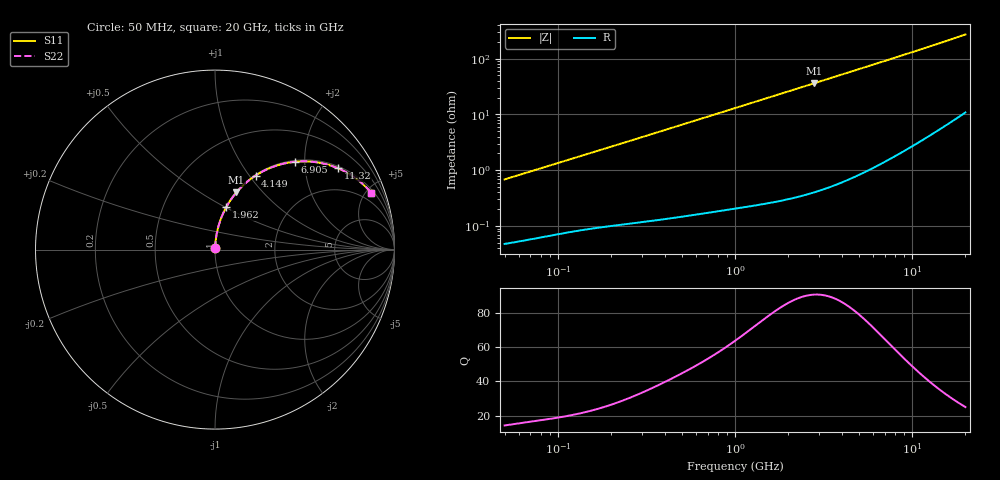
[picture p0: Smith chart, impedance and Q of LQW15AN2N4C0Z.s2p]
!Murata Part Number: LQW15AN2N4C0Z
!These Parameters are Measured in Series Mode Connection
!  o--[Z]--o
!Port1  Port2
!  o-------o
!Freq. Start=50[MHz] Stop=20[GHz], 401[Steps]
# Hz S RI R 50
!Freq.(Hz) S11(Real) S11(Imag) S21(Real) S21(Imag) S12(Real) S12(Imag) S22(Real) S22(Imag)
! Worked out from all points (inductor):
!   401 points, 50 MHz to 20 GHz, reference 50 ohm
!   read as one part in series: L = 2.16 nH near 51.52 MHz
!   highest Q = 90.4 at 2.811 GHz (marker M1), where L = 2.06 nH
!   S11 on the Smith chart (normalised r, x): 50 MHz: 1.00, +0.01; 1.962 GHz: 1.01, +0.51; 4.149 GHz: 1.01, +1.07; 6.905 GHz: 1.03, +1.79; 11.32 GHz: 1.07, +2.97; 20 GHz: 1.22, +5.43
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5e7  0.000523 0.00682  0.9995 -0.00682  0.9995 -0.00682  0.000523 0.00682
5.152053e7  0.000533 0.00703  0.9995 -0.00703  0.9995 -0.00703  0.000533 0.00703
1.364002e8  0.00117 0.0181  0.9988 -0.0181  0.9988 -0.0181  0.00117 0.0181
2.33884e8  0.00201 0.0307  0.998 -0.0307  0.998 -0.0307  0.00201 0.0307
3.721004e8  0.00364 0.0485  0.9964 -0.0485  0.9964 -0.0485  0.00364 0.0485
6.285508e8  0.00825 0.081  0.9918 -0.081  0.9918 -0.081  0.00825 0.081
1e9  0.0185 0.1271  0.9815 -0.1271  0.9815 -0.1271  0.0185 0.1271
1.411297e9  0.0345 0.1761  0.9655 -0.1761  0.9655 -0.1761  0.0345 0.1761
1.962148e9  0.063 0.2372  0.937 -0.2372  0.937 -0.2372  0.063 0.2372
2.728004e9  0.1134 0.3116  0.8866 -0.3116  0.8866 -0.3116  0.1134 0.3116
2.810964e9  0.1195 0.3189  0.8805 -0.3189  0.8805 -0.3189  0.1195 0.3189
3.415248e9  0.1661 0.3667  0.8339 -0.3667  0.8339 -0.3667  0.1661 0.3667
4.149438e9  0.2266 0.4128  0.7734 -0.4128  0.7734 -0.4128  0.2266 0.4128
5.433528e9  0.3337 0.465  0.6663 -0.465  0.6663 -0.465  0.3337 0.465
6.905011e9  0.4467 0.4896  0.5533 -0.4896  0.5533 -0.4896  0.4467 0.4896
7.442007e9  0.4839 0.4917  0.5161 -0.4917  0.5161 -0.4917  0.4839 0.4917
9.178299e9  0.5877 0.4828  0.4123 -0.4828  0.4123 -0.4828  0.5877 0.4828
1.131968e10  0.6843 0.4535  0.3157 -0.4535  0.3157 -0.4535  0.6843 0.4535
1.314879e10  0.7452 0.4228  0.2548 -0.4228  0.2548 -0.4228  0.7452 0.4228
1.527346e10  0.7978 0.3868  0.2022 -0.3868  0.2022 -0.3868  0.7978 0.3868
1.774144e10  0.8419 0.3477  0.1581 -0.3477  0.1581 -0.3477  0.8419 0.3477
2e10  0.8712 0.3156  0.1288 -0.3156  0.1288 -0.3156  0.8712 0.3156
